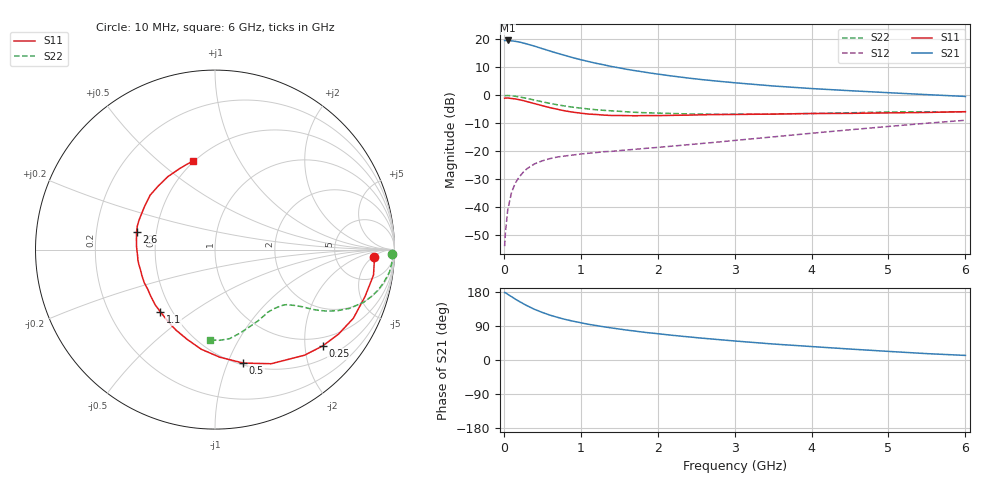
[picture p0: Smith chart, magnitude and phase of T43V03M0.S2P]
! Infineon Technologies  Discrete & RF Semiconductors
! BFR182T
! Si NPN RF Bipolar Junction Transistor in SC75
! VCE = 3 V  IC = 3 mA
! Common Emitter S-Parameters:  October  1999
# GHz  S  MA  R  50
!  f  S11  S21  S12  S22
! GHz  MAG  ANG  MAG  ANG  MAG  ANG  MAG  ANG
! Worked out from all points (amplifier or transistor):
!   36 points, 10 MHz to 6 GHz, reference 50 ohm
!   highest |S21| = 19.6 dB at 50 MHz (marker M1)
!   |S21| within 3 dB of that: start of sweep to 508.8 MHz
!   unconditionally stable (mu >= 1): 1.709 GHz to 4.189 GHz
!   at 250 MHz: K = 0.19, MSG = 23.1 dB, |S12| = -27.6 dB
!   at 1.4 GHz: K = 0.90, MSG = 15.2 dB, |S12| = -20.1 dB
!   at 6 GHz: K = 0.83, MSG = 4.3 dB, |S12| = -8.9 dB
!   lowest NFmin = 1.10 dB at 450 MHz
!   S11 on the Smith chart (normalised r, x): 10 MHz: 14, -6; 250 MHz: 0.78, -2.39; 500 MHz: 0.52, -1.14; 1.1 GHz: 0.43, -0.38; 2.6 GHz: 0.39, +0.10; 6 GHz: 0.49, +0.65
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0.01  0.8849 -2.8  9.541 178.0  0.002 83.2  0.988 -1.5
0.02  0.8898 -2.2  9.49 177.7  0.0034 95.4  0.9855 -1.5
0.05  0.8945 -9.1  9.561 173.4  0.0088 86.6  0.9899 -3.8
0.1  0.876 -17.3  9.41 167.2  0.0183 82.1  0.9799 -7.4
0.15  0.8605 -26.4  9.22 160.6  0.0271 76.8  0.9587 -10.9
0.2  0.8338 -34.4  8.961 154.6  0.0345 72.9  0.936 -14.0
0.25  0.8047 -41.9  8.623 148.9  0.0418 68.0  0.9072 -16.9
0.3  0.7714 -49.7  8.263 143.4  0.0485 65.0  0.8801 -19.4
0.4  0.7087 -63.8  7.554 133.6  0.0594 59.0  0.8183 -23.6
0.5  0.6516 -76.0  6.828 125.5  0.0672 55.0  0.7645 -26.4
0.6  0.5999 -87.5  6.183 118.3  0.0737 51.6  0.7161 -28.6
0.8  0.5241 -107.1  5.138 107.0  0.0823 47.6  0.6404 -31.4
0.9  0.4981 -116.0  4.695 102.4  0.0855 46.7  0.6109 -32.3
1.1  0.461 -131.3  4.017 94.2  0.0919 46.2  0.5688 -33.8
1.3  0.442 -144.2  3.502 87.6  0.098 46.3  0.5376 -35.3
1.6  0.4323 -160.2  2.912 78.9  0.1053 47.6  0.5056 -37.3
2.2  0.4375 177.8  2.197 65.0  0.1235 52.1  0.4719 -43.1
2.6  0.4483 167.1  1.892 57.2  0.1383 55.0  0.4597 -47.8
3.5  0.4603 148.5  1.467 42.2  0.1802 58.7  0.464 -59.3
4.5  0.4747 131.9  1.207 28.9  0.2414 58.9  0.486 -73.5
5.5  0.4931 113.2  1.027 16.8  0.3163 55.5  0.506 -87.0
6  0.5089 104.2  0.953 12.1  0.3574 52.4  0.5033 -92.9
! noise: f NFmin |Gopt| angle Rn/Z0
0.45  1.1  0.37  30  0.33
0.9  1.2  0.35  61  0.26
1.8  1.85  0.27  133  0.2
